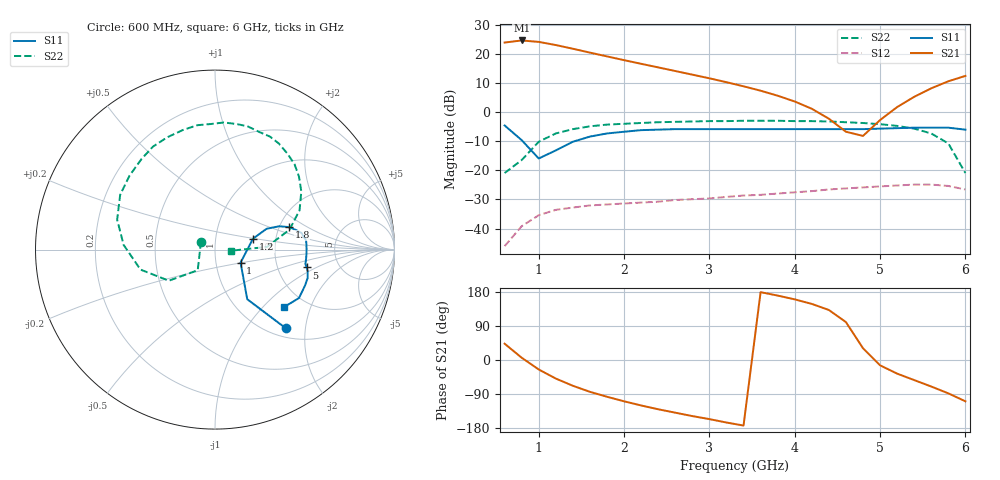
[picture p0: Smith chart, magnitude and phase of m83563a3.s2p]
!	MGA-83563 S PARAMETERS
!	Vd = 3 V L=18 nH  LAST UPDATED 10-15-97
# ghz	s ma r	50
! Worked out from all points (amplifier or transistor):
!   28 points, 600 MHz to 6 GHz, reference 50 ohm
!   highest |S21| = 24.6 dB at 800 MHz (marker M1)
!   |S21| within 3 dB of that: start of sweep to 1.423 GHz
!   unconditionally stable (mu >= 1): start of sweep to end of sweep
!   at 1.4 GHz: K = 1.48, MAG = 23.2 dB, |S12| = -32.8 dB
!   at 3.4 GHz: K = 2.12, MAG = 12.7 dB, |S12| = -28.6 dB
!   at 6 GHz: K = 1.99, MAG = 13.8 dB, |S12| = -26.6 dB
!   S11 on the Smith chart (normalised r, x): 600 MHz: 1.17, -1.57; 1 GHz: 1.32, -0.20; 1.2 GHz: 1.52, +0.19; 1.8 GHz: 2.25, +0.69; 5 GHz: 2.92, -0.80; 6 GHz: 1.55, -1.33
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0.6  0.59 -48.0  15.61 43.0  0.005 105.0  0.09 150.0
0.8  0.33 -57.0  16.96 6.0  0.011 102.0  0.15 -130.0
1  0.16 -27.0  16.02 -25.0  0.017 87.0  0.31 -146.0
1.2  0.22 16.0  14.15 -49.0  0.021 75.0  0.43 -165.0
1.4  0.31 22.0  12.22 -68.0  0.023 66.0  0.51 177.0
1.6  0.38 20.0  10.49 -84.0  0.025 59.0  0.57 163.0
1.8  0.43 17.0  9.03 -97.0  0.026 54.0  0.61 150.0
2  0.46 14.0  7.79 -109.0  0.027 51.0  0.63 139.0
2.2  0.49 11.0  6.74 -120.0  0.028 48.0  0.65 129.0
2.4  0.5 8.0  5.85 -130.0  0.029 46.0  0.67 121.0
2.8  0.51 4.0  4.39 -148.0  0.032 43.0  0.69 105.0
3.2  0.51 1.0  3.26 -165.0  0.035 40.0  0.7 92.0
3.4  0.51 -1.0  2.77 -173.0  0.037 38.0  0.71 86.0
3.8  0.51 -3.0  1.91 170.0  0.04 35.0  0.71 75.0
4.2  0.51 -6.0  1.14 148.0  0.044 31.0  0.7 64.0
4.8  0.51 -9.0  0.39 31.0  0.051 22.0  0.65 47.0
5  0.52 -11.0  0.73 -14.0  0.053 18.0  0.62 41.0
5.2  0.53 -13.0  1.22 -36.0  0.055 13.0  0.58 34.0
5.4  0.54 -17.0  1.83 -53.0  0.057 7.0  0.52 25.0
5.6  0.54 -22.0  2.56 -70.0  0.057 0.0  0.43 15.0
5.8  0.54 -30.0  3.38 -88.0  0.054 -8.0  0.29 3.0
6  0.5 -40.0  4.18 -109.0  0.047 -17.0  0.09 -4.0
